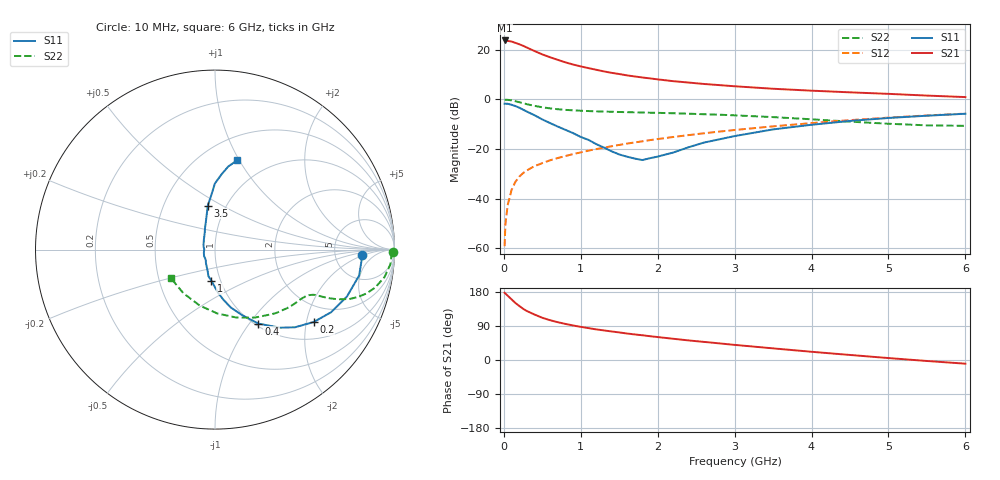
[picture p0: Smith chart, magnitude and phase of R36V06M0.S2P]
! SIEMENS Small Signal Semiconductors
! BFR181
! Si NPN RF Bipolar Junction Transistor in SOT23
! VCE = 6 V  IC = 6 mA
! Common Emitter S-Parameters:  May  1996
# GHz  S  MA  R  50
!  f  S11  S21  S12  S22
! GHz  MAG  ANG  MAG  ANG  MAG  ANG  MAG  ANG
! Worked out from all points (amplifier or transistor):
!   36 points, 10 MHz to 6 GHz, reference 50 ohm
!   highest |S21| = 23.8 dB at 10 MHz (marker M1)
!   |S21| within 3 dB of that: start of sweep to 309.2 MHz
!   unconditionally stable (mu >= 1): 1.11 GHz to 2.94 GHz
!   at 250 MHz: K = 0.45, MSG = 25.7 dB, |S12| = -29.7 dB
!   at 1.4 GHz: K = 1.04, MAG = 13.6 dB, |S12| = -18.9 dB
!   at 6 GHz: K = 0.86, MSG = 3.3 dB, |S12| = -5.7 dB
!   S11 on the Smith chart (normalised r, x): 10 MHz: 10, -2; 200 MHz: 1.46, -2.21; 400 MHz: 1.04, -1.11; 1 GHz: 0.91, -0.32; 3.5 GHz: 0.82, +0.43; 6 GHz: 0.73, +0.98
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0.01  0.821 -2.0  15.43 177.4  0.0011 91.5  0.9911 -0.9
0.02  0.819 -4.1  15.29 175.3  0.003 89.1  0.9837 -2.0
0.05  0.8159 -10.2  15.11 169.7  0.0074 85.2  0.9809 -4.8
0.1  0.7802 -19.6  14.68 160.1  0.0149 80.3  0.9567 -9.2
0.15  0.7346 -28.4  13.8 150.4  0.0218 75.4  0.9187 -13.2
0.2  0.6817 -36.3  12.95 142.7  0.0276 72.5  0.8798 -16.1
0.25  0.6217 -44.1  12.06 135.2  0.0327 69.8  0.8396 -18.3
0.3  0.5673 -50.1  11.09 129.1  0.0371 67.8  0.8003 -20.1
0.4  0.4783 -59.6  9.426 119.9  0.0453 65.7  0.74 -22.0
0.5  0.3945 -67.6  8.071 111.4  0.0519 65.3  0.6941 -23.0
0.6  0.3337 -74.8  7.085 105.1  0.0592 65.2  0.6592 -23.6
0.7  0.2838 -80.4  6.283 99.8  0.0657 65.5  0.6338 -24.0
0.8  0.2436 -85.6  5.588 95.2  0.0722 65.2  0.6151 -24.3
1  0.1747 -96.6  4.628 87.5  0.0855 65.6  0.5914 -25.3
1.1  0.153 -103.8  4.273 84.2  0.0927 65.7  0.5825 -25.8
1.3  0.1072 -115.4  3.669 78.1  0.1065 65.8  0.5681 -27.2
1.6  0.0701 -150.7  3.054 69.9  0.1285 65.5  0.553 -29.8
2.2  0.0848 136.7  2.333 56.1  0.1746 63.2  0.5258 -36.9
3.5  0.2485 99.3  1.639 30.7  0.2863 53.9  0.4396 -59.5
4.5  0.3684 90.1  1.388 13.3  0.3818 43.7  0.3565 -87.8
5.5  0.4693 80.9  1.194 -2.6  0.475 31.3  0.3 -126.0
6  0.5142 75.9  1.114 -9.7  0.5173 24.3  0.293 -147.4
